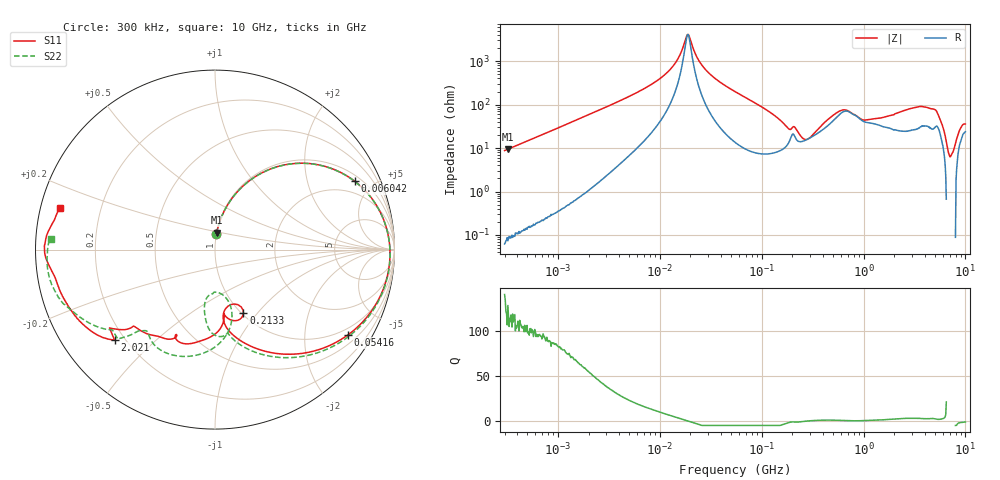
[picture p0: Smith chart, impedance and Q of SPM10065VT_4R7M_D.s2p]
! S-Parameter Data Generated by TDK Corporation
! Copyright(C) 2020 TDK Corporation.
! All Rights Reserved.
! TDK P/N: SPM10065VT-4R7M-D (Inductor)
! Property: L=4.7uH at 100kHz
! Size(LxWxT): 10.5x10x6.5mm
! Model Type: s2p (Touchstone File Format Version 1.0)
! Frequency: DC=Yes Start=0.3MHz Stop=10000MHz 802points Log-sweep
! Model Generated on Apr. 23, 2020
! Port Assignments:
!  1 ---@@@--- 2
! Applicable Conditions:
!  Temperature = 25 degC
!  DC Bias Current = 0 A
!  Small Signal Operation
! Terms and conditions regarding TDK Simulation Models
! (1)This simulation model is being provided solely for informational purposes. Please refer to the specifications of the products in terms of detailed characteristics of such products.
! (2)In no event shall TDK Corporation of any of its subsidiaries be liable for any loss or damage arising, directly or indirectly,
!  From any information contained in this simulation model, including, but not limited to loss or damages arising from any inaccuracies, omissions or errors in connection with such information.
! (3)Any and all copyrights on this simulation model are owned by TDK Corporation.
!  Duplication or redistribution of this simulation model without prior written permission from TDK Corporation is prohibited.
! (4)This simulation model is subject to any modification or change without any prior notice.
! (5)Neither TDK Corporation nor any of its subsidiaries shall make any warranty, express or implied,
!  Including but not limited to the correctness, implied warranties of merchantability and fitness for a particular purpose with respect to this simulation models.
! (6)The use of this simulation model shall be deemed to have consented to the terms and conditions hereof.
# Hz S MA R 50
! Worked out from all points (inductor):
!   801 points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, 300 kHz to 10 GHz, reference 50 ohm
!   read as one part in series: L = 4.62 uH near 318.3 kHz
!   highest Q = 119 at 322.9 kHz (marker M1), where L = 4.64 uH
!   self-resonance near 18.9 MHz
!   S11 on the Smith chart (normalised r, x): 300 kHz: 1.00, +0.18; 6.042 MHz: 1.28, +3.94; 54.16 MHz: 0.77, -3.25; 213.3 MHz: 1.02, -0.85; 2.021 GHz: 0.16, -0.38; 10 GHz: 0.06, +0.13
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300000  0.08791 85.1  0.9948 -4.9  0.9953 -5.0  0.08768 84.9
322921  0.09421 84.6  0.9943 -5.3  0.9947 -5.4  0.09412 84.3
1713600  0.4409 62.7  0.8906 -26.4  0.8903 -26.4  0.441 62.6
6041662  0.8674 26.0  0.4529 -61.0  0.4527 -61.0  0.8678 25.8
9671944  0.9425 13.2  0.2544 -71.4  0.2543 -71.4  0.9429 13.0
1.405002e7  0.9694 4.2  0.1116 -73.6  0.1116 -73.6  0.97 3.8
1.899897e7  0.9756 -2.9  0.02376 1.7  0.02375 1.6  0.9763 -3.5
2.819857e7  0.9643 -12.7  0.1507 67.8  0.1507 67.8  0.9651 -13.5
5.416364e7  0.8804 -32.6  0.4171 52.8  0.417 52.8  0.8817 -34.2
5.477226e7  0.878 -33.0  0.4219 52.5  0.4218 52.5  0.8793 -34.6
1.00316e8  0.6961 -56.8  0.6677 27.9  0.6674 27.9  0.6976 -59.4
1.788252e8  0.4255 -82.3  0.7871 -3.2  0.7868 -3.2  0.4748 -80.9
2.133243e8  0.3884 -65.9  0.7407 -6.9  0.7404 -6.9  0.4633 -92.3
3.126428e8  0.3647 -82.0  0.7814 -30.7  0.7811 -30.7  0.2922 -100.6
4.388767e8  0.3896 -82.6  0.6625 -55.3  0.6623 -55.3  0.2415 -85.1
5.99416e8  0.5039 -96.4  0.4344 -71.3  0.4343 -71.3  0.4296 -78.2
7.497801e8  0.5475 -112.8  0.3728 -68.3  0.3727 -68.3  0.5919 -98.8
9.789263e8  0.5739 -121.8  0.4058 -80.1  0.4057 -80.1  0.6275 -123.1
1.767019e9  0.679 -138.9  0.2341 -146.1  0.234 -146.1  0.6797 -135.1
2.020878e9  0.753 -138.0  0.1787 -162.5  0.1785 -162.5  0.726 -142.0
5.040844e9  0.9039 -170.1  0.01649 173.0  0.01651 173.8  0.9189 -165.0
1e10  0.8952 164.8  0.01979 142.2  0.01979 142.3  0.9159 176.4
